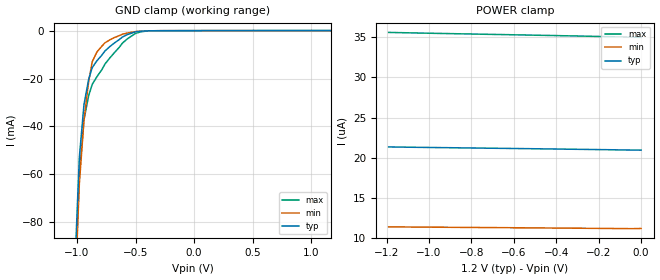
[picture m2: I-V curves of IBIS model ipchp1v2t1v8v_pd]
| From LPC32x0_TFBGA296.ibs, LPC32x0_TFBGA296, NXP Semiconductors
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| |   Rev 0.20 IBIS Model Design Automation Generation   |
| |   N O N - S I L I C O N   C O R R E L A T E D   |
| |   This IBIS [Model] is pre-Beta tactical support   |
| |  Note: this IBIS [Model] contains clamp curves generated   |
| |   through simulation which should not be relied upon   |
| ipchp1v2t1v8v
|   Input Pad 1v2
|   Push Pull
|   CMOS
|   Programmable between
|   - (p1=0, p2=1) plain input
|   - (p1=0, p2=0) with Pull Up
|   - (p1=1, p2=1) with Pull Down
|   - (p1=1, p2=0) with Repeater
|   Characterized at Core 1.2V and I/O 1.8V
| Pull Down Mode (p1=1, p2=1)
[Model]   ipchp1v2t1v8v_pd | of ipchp1v2t1v8v
Model_type   Input
|  Reciever Thresholds
Vinl   = 0.36V
Vinh   = 0.84V
| [Process Range]   typical   min   max
| C_comp edge width   400.000ps   400.000ps   400.000ps
| C_comp Tstrobe   40.000fs   40.000fs   40.000fs
C_comp   2.019pF   1.888pF   2.187pF
[Temperature Range]   25   105   -20
[Voltage Range]   1.20V   1.10V   1.30V
[GND Clamp Reference]   0.00V   0.00V   0.00V
[Pulldown Reference]   0.00V   0.00V   0.00V
[POWER Clamp Reference]   1.20V   1.10V   1.30V
[Pullup Reference]   1.20V   1.10V   1.30V
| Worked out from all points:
|   GND clamp passes 1 mA (typ) near -0.53 V on its own axis
[GND Clamp]
| ref voltage   0.00V   0.00V   0.00V
|   Voltage   I(typ)   I(min)   I(max)
-1.2V     -373.8mA   -377.3mA   -396.4mA
-1.01V    -89.19mA   -101.8mA   -99.48mA
-980mV    -53.07mA   -64.23mA   -60.47mA
-940mV    -30.85mA   -37.28mA   -37.23mA
-900mV    -20.3mA    -21.21mA   -27.11mA
-870mV    -15.47mA   -13mA      -22.46mA
-830mV    -12.6mA    -8.915mA   -19.26mA
-760mV    -8.431mA   -5.043mA   -13.88mA
-570mV    -1.655mA   -988uA     -3.435mA
-500mV    -508.1uA   -391.7uA   -1.156mA
-420mV    -133.8uA   -139.1uA   -246.8uA
1.17V     20.92uA    11.16uA    34.92uA
[Power Clamp]   | Vtable = Vcc - Vpad
| ref voltage   1.20V   1.10V   1.30V
|   Voltage   I(typ)   I(min)   I(max)
-1.19V    21.34uA    11.38uA    35.62uA
-1.15V    21.33uA    11.37uA    35.6uA
-970mV    21.27uA    11.34uA    35.5uA
-410mV    21.09uA    11.23uA    35.23uA
-380mV    21.07uA    11.22uA    35.21uA
-260mV    21.03uA    11.2uA     35.15uA
-230mV    21.02uA    11.2uA     35.13uA
-150mV    21uA       11.18uA    35.09uA
-120mV    20.98uA    11.17uA    35.07uA
-80mV     20.97uA    11.16uA    35.05uA
-40mV     20.95uA    11.15uA    35.03uA
0V        20.94uA    11.18uA    35uA
